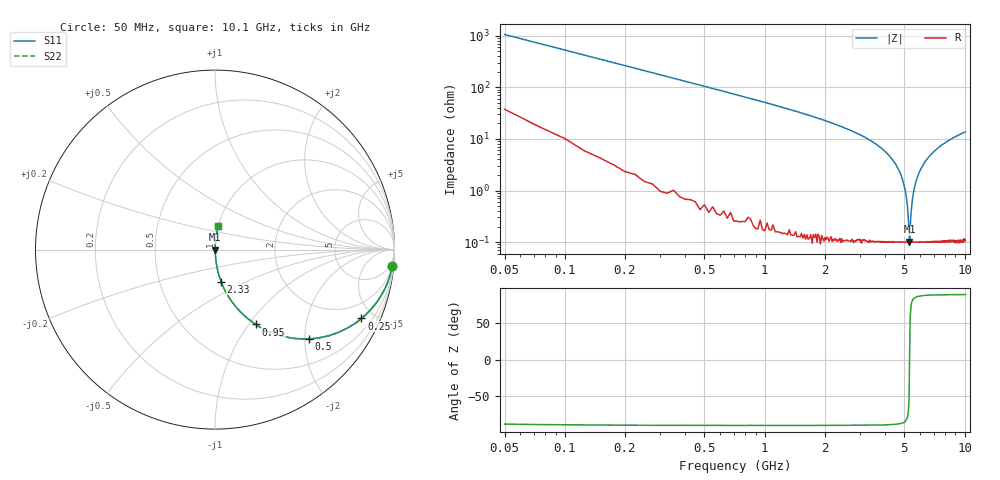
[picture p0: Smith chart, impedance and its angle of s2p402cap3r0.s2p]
! AVX Thin Film Operation		Date: April 2003
! Description: Accu-P® Series, Thin Film, SMD, RF Capacitor
! Part Number: 0402YJ3R0ABW
! 50 MHz  -  10.05 GHz
! Serial Measurements
# hz S db R 50
!	S11		S21		S12		S22
!	dB	Phase	dB	Phase	dB	Phase	dB	Phase
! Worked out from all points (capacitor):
!   400 points, 50 MHz to 10.1 GHz, reference 50 ohm
!   read as one part in series: C = 3 pF near 100 MHz
!   lowest |Z| = 102 mohm at 5.3 GHz (marker M1)
!   series resonance near 5.306 GHz, so ESL is about 300 pH
!   S11 on the Smith chart (normalised r, x): 50 MHz: 2, -21; 250 MHz: 1.03, -4.23; 500 MHz: 1.01, -2.10; 950 MHz: 1.00, -1.08; 2.33 GHz: 1.00, -0.37; 10.1 GHz: 1.00, +0.27
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5e7  -0.07 -5.4  -20.60 82.6  -20.60 82.6  -0.07 -5.4
1.25e8  -0.26 -13.2  -12.80 76.0  -12.80 76.0  -0.26 -13.2
2.5e8  -0.90 -25.2  -7.42 64.4  -7.42 64.4  -0.90 -25.2
5e8  -2.82 -43.4  -3.25 46.3  -3.25 46.3  -2.82 -43.4
9.5e8  -6.47 -61.4  -1.13 28.3  -1.13 28.3  -6.47 -61.4
1.73e9  -11.50 -74.4  -0.33 15.4  -0.33 15.4  -11.50 -74.4
2.33e9  -14.80 -79.2  -0.15 10.4  -0.15 10.4  -14.80 -79.2
3.4e9  -20.80 -84.1  -0.05 5.2  -0.05 5.2  -20.80 -84.1
4.58e9  -30.50 -86.4  -0.01 1.7  -0.01 1.7  -30.50 -86.4
4.88e9  -35.40 -85.6  -0.01 1.0  -0.01 1.0  -35.40 -85.6
5.08e9  -41.00 -83.1  -0.01 0.5  -0.01 0.5  -41.00 -83.1
5.23e9  -49.90 -71.6  -0.01 0.2  -0.01 0.2  -49.90 -71.6
5.3e9  -59.80 -11.0  -0.01 0.0  -0.01 0.0  -59.80 -11.0
5.33e9  -58.10 36.7  -0.01 -0.0  -0.01 -0.0  -58.10 36.7
5.35e9  -54.20 59.2  -0.01 -0.1  -0.01 -0.1  -54.20 59.2
5.4e9  -48.70 74.0  -0.01 -0.2  -0.01 -0.2  -48.70 74.0
5.45e9  -45.20 79.2  -0.01 -0.3  -0.01 -0.3  -45.20 79.2
5.7e9  -36.80 85.2  -0.01 -0.8  -0.01 -0.8  -36.80 85.2
6.08e9  -31.30 86.3  -0.01 -1.6  -0.01 -1.6  -31.30 86.3
6.75e9  -26.30 86.0  -0.02 -2.8  -0.02 -2.8  -26.30 86.0
8.43e9  -20.40 83.9  -0.05 -5.5  -0.05 -5.5  -20.40 83.9
1.01e10  -17.40 81.8  -0.09 -7.8  -0.09 -7.8  -17.40 81.8
